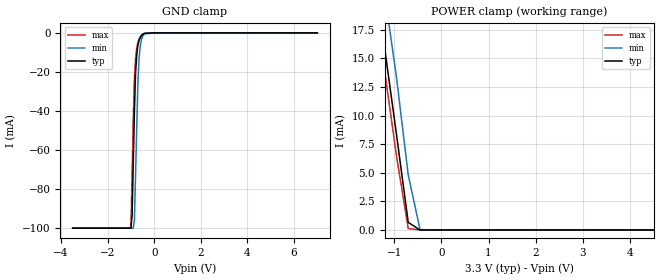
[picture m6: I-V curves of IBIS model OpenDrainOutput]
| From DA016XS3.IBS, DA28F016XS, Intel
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|*****************Open Drain Output Model********************************
[Model]   OpenDrainOutput
Model_type   Open_drain
|   for RY/BY# pin 53
Vinl = 0.8V
Vinh = 2.0V
| Variable   typ   min   max
C_comp   9.61p   NA   11.6p
[Voltage Range]   3.3V   3.0V   3.6V
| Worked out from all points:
|   GND clamp passes 1 mA (typ) near -0.51 V on its own axis
|   POWER clamp passes 1 mA (typ) near -0.71 V on its own axis
[Pulldown]
| [Pullup] and [Pulldown] IV curves include only the current through
| the channels of output driver transistors when outputs are enabled
| with OE# = VIL.  Although the output driver transistors have np and
| pn diodes inherently created by CMOS IC fabrication between the
| drain and bulk of n-channel and p-channel CMOS transistors,
| the current through these junction diodes is not included in
| [Pullup] or [Pulldown].  Instead that drain/bulk diode current is
| included in the [POWER_clamp] or [GND_clamp] sections, which are
| not dependent on the state of OE# or output data value.  The RY/BY#
| Pulldown information is not provided for this device.  The table
| below is for the compatibility with some IBIS parsers.
|Voltage  I(typ)   I(min)   I(max)
-3.5V     0A         0A         0A
6.75V     0A         0A         0A
[GND_clamp]
| [POWER_clamp] and [GND_clamp] IV curves describe ESD protection
| circuits PLUS some np and pn diodes which exist between the
| drain and bulk of n-channel and p-channel CMOS transistors.
| These drain/bulk diodes are inherent in CMOS IC fabrication,
| and are visible on the node of the I/O pin at all times.
| Even the drain/bulk diodes of output driver [Pullup] and [Powerdown]
| transistors are included in [POWER_clamp] or [GND_clamp], because
| these diodes contribute to I/O pin current even when the
| chip outputs are tristated by OE# = VIH.
|Voltage  I(typ)   I(min)   I(max)
-3.5V     -99.95mA   -99.93mA   -99.95mA
-1V       -99.95mA   -99.93mA   -99.95mA
-950mV    -93.51mA   -99.93mA   -71.83mA
-900mV    -66.68mA   -99.93mA   -44.02mA
-850mV    -39.77mA   -95.97mA   -22.77mA
-800mV    -20.07mA   -71.95mA   -12.93mA
-750mV    -11.12mA   -47.78mA   -7.498mA
-700mV    -6.24mA    -25.47mA   -4.787mA
-650mV    -3.793mA   -12.62mA   -3.189mA
-600mV    -2.386mA   -6.702mA   -2.063mA
-500mV    -839.6uA   -1.846mA   -679.8uA
7V        0A         0A         0A
[Pullup]
| (Voltages for [Pullup] and [POWER_clamp] are specified with
| negative respect to Vcc.  Reference the IBIS documentation
| for more information regarding Vtable = Vcc - Voutput.
| This method keeps -Vds constant for the values in all three
| columns across a line of the table.)
| [Pullup] and [Pulldown] IV curves include only the current through
| the channels of output driver transistors when outputs are enabled
| with OE# = VIL.  Although the output driver transistors have np and
| pn diodes inherently created by CMOS IC fabrication between the
| drain and bulk of n-channel and p-channel CMOS transistors,
| the current through these junction diodes is not included in
| [Pullup] or [Pulldown].  Instead that drain/bulk diode current is
| included in the [POWER_clamp] or [GND_clamp] sections, which are
| not dependent on the state of OE# or output data value.
|Voltage  I(typ)   I(min)   I(max)
-3.5V     0A         0A         0A
6.75V     0A         0A         0A
[POWER_clamp]
| (Voltages for [Pullup] and [POWER_clamp] are specified with
| negative respect to Vcc.  Reference the IBIS documentation
| for more information regarding Vtable = Vcc - Voutput.
| This method keeps -Vds constant for the values in all three
| columns across a line of the table. For example, on the seventh
| line of the table below, Voltage = -2V on this 3.3V+-10% VCC model
| means Voutput with respect to ground is forced to about 5.3(typ),
| 5.0V (min), and 5.6V (max), and in all three cases -Vds = -2V.)
| [POWER_clamp] and [GND_clamp] IV curves describe ESD protection
| circuits PLUS some np and pn diodes which exist between the
| drain and bulk of n-channel and p-channel CMOS transistors.
| These drain/bulk diodes are inherent in CMOS IC fabrication,
| and are visible on the node of the I/O pin at all times.
| Even the drain/bulk diodes of output driver [Pullup] and [Powerdown]
| transistors are included in [POWER_clamp] or [GND_clamp], because
| these diodes contribute to I/O pin current even when the
| chip outputs are tristated by OE# = VIH.
| For example, when V forced on the I/O pin is large, we are
| forward biasing the pn diode at the drain/bulk interface in the
| p-channel pullup transistor.  Similarly, when V forced on the
| I/O pin is sufficiently negative with respect to the substrate
| ground, we are forward biasing the np diode at the drain/bulk
| interface in the n-channel pulldown transistor.  The effects
| of these diodes are included in [POWER_clamp] or [GND_clamp].
|Voltage  I(typ)   I(min)   I(max)
-3.7V     73.37mA    74.55mA    72.53mA
-1.45V    22.48mA    27.02mA    20.46mA
-1.2V     15.91mA    20.67mA    13.93mA
-950mV    8.383mA    13.38mA    6.49mA
-700mV    657uA      4.804mA    121.6uA
-450mV    0A         35.86uA    0A
6.8V      0A         0A         0A
[Ramp]
| The RY/BY# Ramp information is not provided for this device.  The table
| below is for the compatibility with some IBIS parsers.
| Variable   typ   min   max
 dV/dt_r   0V/0ns   0V/0ns   0V/0ns
 dV/dt_f   0V/0ns   0V/0ns   0V/0ns
